|   stm32f401_b_c_lqfp64 IBIS Model
[IBIS ver]   4.2
[File name]  stm32f401_b_c_lqfp64.ibs
[File Rev]   1.0
[Date]   09-06-2015
[Source] Data Created at STMicroelectronics
[Notes]   File originated from ELDO simulations.
[Disclaimer]  This information is for modeling purpose only and is
   not guaranted. The information is subject to change without
   notice.
[Copyright] Copyright 2015 STMicroelectronics Inc.
[Component] stm32f401_b_c_lqfp64
[Manufacturer] STMicroelectronics
[Package]
| variable   typ   min   max
R_pkg   0.0   NA   NA
L_pkg   0.0H   NA   NA
C_pkg   0.0F   NA   NA
[Pin]   signal_name   model_name   R_pin   L_pin   C_pin
1 VBAT POWER 63.756E-3 3.679E-9 93.469E-15
2 PC13-ANTI_TAMP io8p_arwsudq_ft_v33 68.980E-3 4.220E-9 120.000E-15
3 PC14-OSC32_IN io8p_arwsudq_ft 59.336E-3 3.221E-9 71.020E-15
4 PC15-OSC32_OUT io8p_arsudq_ft 55.719E-3 2.846E-9 52.653E-15
5 PH0-OSC_IN io8p_arsudq_ft 52.907E-3 2.555E-9 38.367E-15
6 PH1-OSC_OUT io8p_arsudq_ft 50.897E-3 2.347E-9 28.163E-15
7 NRST ioreset_ft_v33 49.692E-3 2.222E-9 22.041E-15
8 PC0 io8p_arwsudq_ft 49.290E-3 2.180E-9 20.000E-15
9 PC1 io8p_arwsudq_ft 49.290E-3 2.180E-9 20.000E-15
10 PC2 io8p_arwsudq_ft 49.692E-3 2.222E-9 22.041E-15
11 PC3 io8p_arwsudq_ft 50.897E-3 2.347E-9 28.163E-15
12 VSSA GND 52.907E-3 2.555E-9 38.367E-15
13 VDDA POWER 55.719E-3 2.846E-9 52.653E-15
14 PA0-WKUP io8p_arwsudq_ft_v33 59.336E-3 3.221E-9 71.020E-15
15 PA1 io8p_arwsudq_ft 63.756E-3 3.679E-9 93.469E-15
16 PA2 io8p_arwsudq_ft 68.980E-3 4.220E-9 120.000E-15
17 PA3 io8p_arwsudq_ft 68.980E-3 4.220E-9 120.000E-15
18 VSS GND 63.756E-3 3.679E-9 93.469E-15
19 VDD POWER 59.336E-3 3.221E-9 71.020E-15
20 PA4 io8p_ar3wsudq_ft 55.719E-3 2.846E-9 52.653E-15
21 PA5 io8p_ar3wsudq_ft 52.907E-3 2.555E-9 38.367E-15
22 PA6 io8p_ar3wsudq_ft 50.897E-3 2.347E-9 28.163E-15
23 PA7 io8p_arwsudq_ft 49.692E-3 2.222E-9 22.041E-15
24 PC4 io8p_arwsudq_ft 49.290E-3 2.180E-9 20.000E-15
25 PC5 io8p_arwsudq_ft 49.290E-3 2.180E-9 20.000E-15
26 PB0 io8p_ar3wsudq_ft 49.692E-3 2.222E-9 22.041E-15
27 PB1 io8p_ar3wsudq_ft 50.897E-3 2.347E-9 28.163E-15
28 PB2 io8p_arwsudq_ft 52.907E-3 2.555E-9 38.367E-15
29 PB10 io8p_arsudq_i2cin_ft 55.719E-3 2.846E-9 52.653E-15
30 VCAP1 POWER 59.336E-3 3.221E-9 71.020E-15
31 VSS GND 63.756E-3 3.679E-9 93.469E-15
32 VDD POWER 68.980E-3 4.220E-9 120.000E-15
33 PB12 io8p_arsudq_ft 68.980E-3 4.220E-9 120.000E-15
34 PB13 io8p_arsudq_ft 63.756E-3 3.679E-9 93.469E-15
35 PB14 io8p_arsudq_ft 59.336E-3 3.221E-9 71.020E-15
36 PB15 io8p_arsudq_ft 55.719E-3 2.846E-9 52.653E-15
37 PC6 io8p_arsudq_ft 52.907E-3 2.555E-9 38.367E-15
38 PC7 io8p_arsudq_ft 50.897E-3 2.347E-9 28.163E-15
39 PC8 io8p_arsudq_ft 49.692E-3 2.222E-9 22.041E-15
40 PC9 io8p_arsudq_i2cin_ft 49.290E-3 2.180E-9 20.000E-15
41 PA8 io8p_arsudq_i2cin_ft 49.290E-3 2.180E-9 20.000E-15
42 PA9 io8usb_vbus_otg_ft 49.692E-3 2.222E-9 22.041E-15
43 PA10 io8usb_id_otg_ft 50.897E-3 2.347E-9 28.163E-15
44 PA11 io8usb_lsfs_otg_ft 52.907E-3 2.555E-9 38.367E-15
45 PA12 io8usb_lsfs_otg_ft 55.719E-3 2.846E-9 52.653E-15
46 PA13 io8p_arsudq_ft 59.336E-3 3.221E-9 71.020E-15
47 VSS GND 63.756E-3 3.679E-9 93.469E-15
48 VDD POWER 68.980E-3 4.220E-9 120.000E-15
49 PA14 io8p_arsudq_ft 68.980E-3 4.220E-9 120.000E-15
50 PA15 io8p_arsudq_ft 63.756E-3 3.679E-9 93.469E-15
51 PC10 io8p_arsudq_ft 59.336E-3 3.221E-9 71.020E-15
52 PC11 io8p_arsudq_ft 55.719E-3 2.846E-9 52.653E-15
53 PC12 io8p_arsudq_ft 52.907E-3 2.555E-9 38.367E-15
54 PD2 io8p_arsudq_ft 50.897E-3 2.347E-9 28.163E-15
55 PB3 io8p_arsudq_i2cin_ft 49.692E-3 2.222E-9 22.041E-15
56 PB4 io8p_arsudq_i2cin_ft 49.290E-3 2.180E-9 20.000E-15
57 PB5 io8p_ar3wsudq_ft 49.290E-3 2.180E-9 20.000E-15
58 PB6 io8p_arsudq_i2cin_ft 49.692E-3 2.222E-9 22.041E-15
59 PB7 io8p_arsudq_i2cin_ft 50.897E-3 2.347E-9 28.163E-15
60 BOOT0 vpp_test_hv 52.907E-3 2.555E-9 38.367E-15
61 PB8 io8p_arsudq_i2cin_ft 55.719E-3 2.846E-9 52.653E-15
62 PB9 io8p_arsudq_i2cin_ft 59.336E-3 3.221E-9 71.020E-15
63 VSS GND 63.756E-3 3.679E-9 93.469E-15
64 VDD POWER 68.980E-3 4.220E-9 120.000E-15
[Diff Pin]   inv_pin   vdiff   tdelay_typ  tdelay_min  tdelay_max
44 45 200mV   NA   NA   NA
[Model Selector] io8p_ar3wsudq_ft
io8p00_ar3wsudq_ft_pd_lv  "SPEED00 1P8V, PD=40kOhm"
io8p00_ar3wsudq_ft_pu_lv  "SPEED00 1P8V, PU=40kOhm"
io8p00_ar3wsudq_ft_lv  "SPEED00 1P8V"
io8p01_ar3wsudq_ft_pd_lv  "SPEED01 1P8V, PD=40kOhm"
io8p01_ar3wsudq_ft_pu_lv  "SPEED01 1P8V, PU=40kOhm"
io8p01_ar3wsudq_ft_lv  "SPEED01 1P8V"
io8p10_ar3wsudq_ft_pd_lv  "SPEED10 1P8V, PD=40kOhm"
io8p10_ar3wsudq_ft_pu_lv  "SPEED10 1P8V, PU=40kOhm"
io8p10_ar3wsudq_ft_lv  "SPEED10 1P8V"
io8p11_ar3wsudq_ft_pd_lv  "SPEED11 1P8V, PD=40kOhm"
io8p11_ar3wsudq_ft_pu_lv  "SPEED11 1P8V, PU=40kOhm"
io8p11_ar3wsudq_ft_lv  "SPEED11 1P8V"
io8p00_ar3wsudq_ft_pd  "SPEED00, PD=40kOhm"
io8p00_ar3wsudq_ft_pu  "SPEED00, PU=40kOhm"
io8p00_ar3wsudq_ft  "SPEED00"
io8p01_ar3wsudq_ft_pd  "SPEED01, PD=40kOhm"
io8p01_ar3wsudq_ft_pu  "SPEED01, PU=40kOhm"
io8p01_ar3wsudq_ft  "SPEED01"
io8p10_ar3wsudq_ft_pd  "SPEED10, PD=40kOhm"
io8p10_ar3wsudq_ft_pu  "SPEED10, PU=40kOhm"
io8p10_ar3wsudq_ft  "SPEED10"
io8p11_ar3wsudq_ft_pd  "SPEED11, PD=40kOhm"
io8p11_ar3wsudq_ft_pu  "SPEED11, PU=40kOhm"
io8p11_ar3wsudq_ft  "SPEED11"
[Model Selector] io8p_arsudq_ft
io8p00_arsudq_ft_pd_lv  "SPEED00 1P8V, PD=40kOhm"
io8p00_arsudq_ft_pu_lv  "SPEED00 1P8V, PU=40kOhm"
io8p00_arsudq_ft_lv  "SPEED00 1P8V"
io8p01_arsudq_ft_pd_lv  "SPEED01 1P8V, PD=40kOhm"
io8p01_arsudq_ft_pu_lv  "SPEED01 1P8V, PU=40kOhm"
io8p01_arsudq_ft_lv  "SPEED01 1P8V"
io8p10_arsudq_ft_pd_lv  "SPEED10 1P8V, PD=40kOhm"
io8p10_arsudq_ft_pu_lv  "SPEED10 1P8V, PU=40kOhm"
io8p10_arsudq_ft_lv  "SPEED10 1P8V"
io8p11_arsudq_ft_pd_lv  "SPEED11 1P8V, PD=40kOhm"
io8p11_arsudq_ft_pu_lv  "SPEED11 1P8V, PU=40kOhm"
io8p11_arsudq_ft_lv  "SPEED11 1P8V"
io8p00_arsudq_ft_pd  "SPEED00, PD=40kOhm"
io8p00_arsudq_ft_pu  "SPEED00, PU=40kOhm"
io8p00_arsudq_ft  "SPEED00"
io8p01_arsudq_ft_pd  "SPEED01, PD=40kOhm"
io8p01_arsudq_ft_pu  "SPEED01, PU=40kOhm"
io8p01_arsudq_ft  "SPEED01"
io8p10_arsudq_ft_pd  "SPEED10, PD=40kOhm"
io8p10_arsudq_ft_pu  "SPEED10, PU=40kOhm"
io8p10_arsudq_ft  "SPEED10"
io8p11_arsudq_ft_pd  "SPEED11, PD=40kOhm"
io8p11_arsudq_ft_pu  "SPEED11, PU=40kOhm"
io8p11_arsudq_ft  "SPEED11"
[Model Selector] io8p_arsudq_i2cin_ft
io8p00_arsudq_i2cin_ft_pd_lv  "SPEED00 1P8V, PD=40kOhm"
io8p00_arsudq_i2cin_ft_pu_lv  "SPEED00 1P8V, PU=40kOhm"
io8p00_arsudq_i2cin_ft_lv  "SPEED00 1P8V"
io8p01_arsudq_i2cin_ft_pd_lv  "SPEED01 1P8V, PD=40kOhm"
io8p01_arsudq_i2cin_ft_pu_lv  "SPEED01 1P8V, PU=40kOhm"
io8p01_arsudq_i2cin_ft_lv  "SPEED01 1P8V"
io8p10_arsudq_i2cin_ft_pd_lv  "SPEED10 1P8V, PD=40kOhm"
io8p10_arsudq_i2cin_ft_pu_lv  "SPEED10 1P8V, PU=40kOhm"
io8p10_arsudq_i2cin_ft_lv  "SPEED10 1P8V"
io8p11_arsudq_i2cin_ft_pd_lv  "SPEED11 1P8V, PD=40kOhm"
io8p11_arsudq_i2cin_ft_pu_lv  "SPEED11 1P8V, PU=40kOhm"
io8p11_arsudq_i2cin_ft_lv  "SPEED11 1P8V"
io8p00_arsudq_i2cin_ft_pd  "SPEED00, PD=40kOhm"
io8p00_arsudq_i2cin_ft_pu  "SPEED00, PU=40kOhm"
io8p00_arsudq_i2cin_ft  "SPEED00"
io8p01_arsudq_i2cin_ft_pd  "SPEED01, PD=40kOhm"
io8p01_arsudq_i2cin_ft_pu  "SPEED01, PU=40kOhm"
io8p01_arsudq_i2cin_ft  "SPEED01"
io8p10_arsudq_i2cin_ft_pd  "SPEED10, PD=40kOhm"
io8p10_arsudq_i2cin_ft_pu  "SPEED10, PU=40kOhm"
io8p10_arsudq_i2cin_ft  "SPEED10"
io8p11_arsudq_i2cin_ft_pd  "SPEED11, PD=40kOhm"
io8p11_arsudq_i2cin_ft_pu  "SPEED11, PU=40kOhm"
io8p11_arsudq_i2cin_ft  "SPEED11"
[Model Selector] io8p_arwsudq_ft
io8p00_arwsudq_ft_pd_lv  "SPEED00 1P8V, PD=40kOhm"
io8p00_arwsudq_ft_pu_lv  "SPEED00 1P8V, PU=40kOhm"
io8p00_arwsudq_ft_lv  "SPEED00 1P8V"
io8p01_arwsudq_ft_pd_lv  "SPEED01 1P8V, PD=40kOhm"
io8p01_arwsudq_ft_pu_lv  "SPEED01 1P8V, PU=40kOhm"
io8p01_arwsudq_ft_lv  "SPEED01 1P8V"
io8p10_arwsudq_ft_pd_lv  "SPEED10 1P8V, PD=40kOhm"
io8p10_arwsudq_ft_pu_lv  "SPEED10 1P8V, PU=40kOhm"
io8p10_arwsudq_ft_lv  "SPEED10 1P8V"
io8p11_arwsudq_ft_pd_lv  "SPEED11 1P8V, PD=40kOhm"
io8p11_arwsudq_ft_pu_lv  "SPEED11 1P8V, PU=40kOhm"
io8p11_arwsudq_ft_lv  "SPEED11 1P8V"
io8p00_arwsudq_ft_pd  "SPEED00, PD=40kOhm"
io8p00_arwsudq_ft_pu  "SPEED00, PU=40kOhm"
io8p00_arwsudq_ft  "SPEED00"
io8p01_arwsudq_ft_pd  "SPEED01, PD=40kOhm"
io8p01_arwsudq_ft_pu  "SPEED01, PU=40kOhm"
io8p01_arwsudq_ft  "SPEED01"
io8p10_arwsudq_ft_pd  "SPEED10, PD=40kOhm"
io8p10_arwsudq_ft_pu  "SPEED10, PU=40kOhm"
io8p10_arwsudq_ft  "SPEED10"
io8p11_arwsudq_ft_pd  "SPEED11, PD=40kOhm"
io8p11_arwsudq_ft_pu  "SPEED11, PU=40kOhm"
io8p11_arwsudq_ft  "SPEED11"
[Model Selector] io8p_arwsudq_ft_v33
io8p00_arwsudq_ft_v33_pd_lv  "SPEED00 1P8V, PD=40kOhm"
io8p00_arwsudq_ft_v33_pu_lv  "SPEED00 1P8V, PU=40kOhm"
io8p00_arwsudq_ft_v33_lv  "SPEED00 1P8V"
io8p01_arwsudq_ft_v33_pd_lv  "SPEED01 1P8V, PD=40kOhm"
io8p01_arwsudq_ft_v33_pu_lv  "SPEED01 1P8V, PU=40kOhm"
io8p01_arwsudq_ft_v33_lv  "SPEED01 1P8V"
io8p10_arwsudq_ft_v33_pd_lv  "SPEED10 1P8V, PD=40kOhm"
io8p10_arwsudq_ft_v33_pu_lv  "SPEED10 1P8V, PU=40kOhm"
io8p10_arwsudq_ft_v33_lv  "SPEED10 1P8V"
io8p11_arwsudq_ft_v33_pd_lv  "SPEED11 1P8V, PD=40kOhm"
io8p11_arwsudq_ft_v33_pu_lv  "SPEED11 1P8V, PU=40kOhm"
io8p11_arwsudq_ft_v33_lv  "SPEED11 1P8V"
io8p00_arwsudq_ft_v33_pd  "SPEED00, PD=40kOhm"
io8p00_arwsudq_ft_v33_pu  "SPEED00, PU=40kOhm"
io8p00_arwsudq_ft_v33  "SPEED00"
io8p01_arwsudq_ft_v33_pd  "SPEED01, PD=40kOhm"
io8p01_arwsudq_ft_v33_pu  "SPEED01, PU=40kOhm"
io8p01_arwsudq_ft_v33  "SPEED01"
io8p10_arwsudq_ft_v33_pd  "SPEED10, PD=40kOhm"
io8p10_arwsudq_ft_v33_pu  "SPEED10, PU=40kOhm"
io8p10_arwsudq_ft_v33  "SPEED10"
io8p11_arwsudq_ft_v33_pd  "SPEED11, PD=40kOhm"
io8p11_arwsudq_ft_v33_pu  "SPEED11, PU=40kOhm"
io8p11_arwsudq_ft_v33  "SPEED11"
[Model Selector] io8usb_id_otg_ft
io8p00_id_otg_ft_pd_lv  "SPEED00 1P8V, PD=14kOhm"
io8p00_id_otg_ft_pu_lv  "SPEED00 1P8V, PU=14kOhm"
io8p00_id_otg_ft_lv  "SPEED00 1P8V"
io8p01_id_otg_ft_pd_lv  "SPEED01 1P8V, PD=14kOhm"
io8p01_id_otg_ft_pu_lv  "SPEED01 1P8V, PU=14kOhm"
io8p01_id_otg_ft_lv  "SPEED01 1P8V"
io8p10_id_otg_ft_pd_lv  "SPEED10 1P8V, PD=14kOhm"
io8p10_id_otg_ft_pu_lv  "SPEED10 1P8V, PU=14kOhm"
io8p10_id_otg_ft_lv  "SPEED10 1P8V"
io8p11_id_otg_ft_pd_lv  "SPEED11 1P8V, PD=14kOhm"
io8p11_id_otg_ft_pu_lv  "SPEED11 1P8V, PU=14kOhm"
io8p11_id_otg_ft_lv  "SPEED11 1P8V"
io8p00_id_otg_ft_pd  "SPEED00, PD=14kOhm"
io8p00_id_otg_ft_pu  "SPEED00, PU=14kOhm"
io8p00_id_otg_ft  "SPEED00"
io8p01_id_otg_ft_pd  "SPEED01, PD=14kOhm"
io8p01_id_otg_ft_pu  "SPEED01, PU=14kOhm"
io8p01_id_otg_ft  "SPEED01"
io8p10_id_otg_ft_pd  "SPEED10, PD=14kOhm"
io8p10_id_otg_ft_pu  "SPEED10, PU=14kOhm"
io8p10_id_otg_ft  "SPEED10"
io8p11_id_otg_ft_pd  "SPEED11, PD=14kOhm"
io8p11_id_otg_ft_pu  "SPEED11, PU=14kOhm"
io8p11_id_otg_ft  "SPEED11"
[Model Selector] io8usb_lsfs_otg_ft
io8usb_ls_otg_ft_dpdn_pd  "LS USB DP/DN IO + PD=20kOhm"
io8usb_ls_otg_ft_dpdn_pupu2  "LS USB DP/DN IO + PU/PU2=2.2kOhm"
io8usb_ls_otg_ft_dpdn_pu2  "LS USB DP/DN IO + PU2=1.2kOhm"
io8usb_ls_otg_ft_dpdn_pu  "LS USB DP/DN IO + PU=1.2kOhm"
io8usb_ls_otg_ft_dpdn  "LS USB DP/DN IO"
io8usb_fs_otg_ft_dpdn_pd  "HS USB DP/DN IO + PD=20kOhm"
io8usb_fs_otg_ft_dpdn_pupu2  "HS USB DP/DN IO + PU/PU2=2.2kOhm"
io8usb_fs_otg_ft_dpdn_pu2  "HS USB DP/DN IO + PU2=1.2kOhm"
io8usb_fs_otg_ft_dpdn_pu  "HS USB DP/DN IO + PU=1.2kOhm"
io8usb_fs_otg_ft_dpdn  "HS USB DP/DN IO"
io8p00_lsfs_otg_ft_pd_lv  "SPEED00 1P8V, PD=40kOhm"
io8p00_lsfs_otg_ft_pu_lv  "SPEED00 1P8V, PU=40kOhm"
io8p00_lsfs_otg_ft_lv  "SPEED00 1P8V"
io8p01_lsfs_otg_ft_pd_lv  "SPEED01 1P8V, PD=40kOhm"
io8p01_lsfs_otg_ft_pu_lv  "SPEED01 1P8V, PU=40kOhm"
io8p01_lsfs_otg_ft_lv  "SPEED01 1P8V"
io8p10_lsfs_otg_ft_pd_lv  "SPEED10 1P8V, PD=40kOhm"
io8p10_lsfs_otg_ft_pu_lv  "SPEED10 1P8V, PU=40kOhm"
io8p10_lsfs_otg_ft_lv  "SPEED10 1P8V"
io8p11_lsfs_otg_ft_pd_lv  "SPEED11 1P8V, PD=40kOhm"
io8p11_lsfs_otg_ft_pu_lv  "SPEED11 1P8V, PU=40kOhm"
io8p11_lsfs_otg_ft_lv  "SPEED11 1P8V"
io8p00_lsfs_otg_ft_pd  "SPEED00, PD=40kOhm"
io8p00_lsfs_otg_ft_pu  "SPEED00, PU=40kOhm"
io8p00_lsfs_otg_ft  "SPEED00"
io8p01_lsfs_otg_ft_pd  "SPEED01, PD=40kOhm"
io8p01_lsfs_otg_ft_pu  "SPEED01, PU=40kOhm"
io8p01_lsfs_otg_ft  "SPEED01"
io8p10_lsfs_otg_ft_pd  "SPEED10, PD=40kOhm"
io8p10_lsfs_otg_ft_pu  "SPEED10, PU=40kOhm"
io8p10_lsfs_otg_ft  "SPEED10"
io8p11_lsfs_otg_ft_pd  "SPEED11, PD=40kOhm"
io8p11_lsfs_otg_ft_pu  "SPEED11, PU=40kOhm"
io8p11_lsfs_otg_ft  "SPEED11"
[Model Selector] io8usb_vbus_otg_ft
io8psenb_vbus_otg_ft  "VBUS PULSE, SENSE VB"
io8psenab_vbus_otg_ft  "VBUS PULSE, SENSE VA and VB"
io8psena_vbus_otg_ft  "VBUS PULSE, SENSE VA"
io8psen_vbus_otg_ft  "VBUS PULSE"
io8p00_vbus_otg_ft_pd_lv  "SPEED00 1P8V, PD=40kOhm"
io8p00_vbus_otg_ft_pu_lv  "SPEED00 1P8V, PU=40kOhm"
io8p00_vbus_otg_ft_lv  "SPEED00 1P8V"
io8p01_vbus_otg_ft_pd_lv  "SPEED01 1P8V, PD=40kOhm"
io8p01_vbus_otg_ft_pu_lv  "SPEED01 1P8V, PU=40kOhm"
io8p01_vbus_otg_ft_lv  "SPEED01 1P8V"
io8p10_vbus_otg_ft_pd_lv  "SPEED10 1P8V, PD=40kOhm"
io8p10_vbus_otg_ft_pu_lv  "SPEED10 1P8V, PU=40kOhm"
io8p10_vbus_otg_ft_lv  "SPEED10 1P8V"
io8p11_vbus_otg_ft_pd_lv  "SPEED11 1P8V, PD=40kOhm"
io8p11_vbus_otg_ft_pu_lv  "SPEED11 1P8V, PU=40kOhm"
io8p11_vbus_otg_ft_lv  "SPEED11 1P8V"
io8p00_vbus_otg_ft_pd  "SPEED00, PD=40kOhm"
io8p00_vbus_otg_ft_pu  "SPEED00, PU=40kOhm"
io8p00_vbus_otg_ft  "SPEED00"
io8p01_vbus_otg_ft_pd  "SPEED01, PD=40kOhm"
io8p01_vbus_otg_ft_pu  "SPEED01, PU=40kOhm"
io8p01_vbus_otg_ft  "SPEED01"
io8p10_vbus_otg_ft_pd  "SPEED10, PD=40kOhm"
io8p10_vbus_otg_ft_pu  "SPEED10, PU=40kOhm"
io8p10_vbus_otg_ft  "SPEED10"
io8p11_vbus_otg_ft_pd  "SPEED11, PD=40kOhm"
io8p11_vbus_otg_ft_pu  "SPEED11, PU=40kOhm"
io8p11_vbus_otg_ft  "SPEED11"
[Model Selector] ioreset_ft_v33
ioreset_ft_v33_pu_lv  "ioreset 1P8V + PU=40kOhm"
ioreset_ft_v33_nopu_lv  "ioreset 1P8V"
ioreset_ft_v33_pu  "ioreset + PU=40kOhm"
ioreset_ft_v33_nopu  "ioreset"
[Model Selector] vpp_test_hv
vpp_test_hv_2p4  "Input Buffer 1P8V"
vpp_test_hv_3p3  "Input Buffer"
| Models and submodels in the file (212): io8p00_ar3wsudq_ft_pd_lv (I/O), io8p00_ar3wsudq_ft_pu_lv (I/O), io8p00_ar3wsudq_ft_lv (I/O), io8p01_ar3wsudq_ft_pd_lv (I/O), io8p01_ar3wsudq_ft_pu_lv (I/O), io8p01_ar3wsudq_ft_lv (I/O), io8p10_ar3wsudq_ft_pd_lv (I/O), io8p10_ar3wsudq_ft_pu_lv (I/O), io8p10_ar3wsudq_ft_lv (I/O), io8p11_ar3wsudq_ft_pd_lv (I/O), io8p11_ar3wsudq_ft_pu_lv (I/O), io8p11_ar3wsudq_ft_lv (I/O), io8p00_ar3wsudq_ft_pd (I/O), io8p00_ar3wsudq_ft_pu (I/O), io8p00_ar3wsudq_ft (I/O), io8p01_ar3wsudq_ft_pd (I/O), io8p01_ar3wsudq_ft_pu (I/O), io8p01_ar3wsudq_ft (I/O), io8p10_ar3wsudq_ft_pd (I/O), io8p10_ar3wsudq_ft_pu (I/O), io8p10_ar3wsudq_ft (I/O), io8p11_ar3wsudq_ft_pd (I/O), io8p11_ar3wsudq_ft_pu (I/O), io8p11_ar3wsudq_ft (I/O), io8p00_arsudq_ft_pd_lv (I/O), io8p00_arsudq_ft_pu_lv (I/O), io8p00_arsudq_ft_lv (I/O), io8p01_arsudq_ft_pd_lv (I/O), io8p01_arsudq_ft_pu_lv (I/O), io8p01_arsudq_ft_lv (I/O), io8p10_arsudq_ft_pd_lv (I/O), io8p10_arsudq_ft_pu_lv (I/O), io8p10_arsudq_ft_lv (I/O), io8p11_arsudq_ft_pd_lv (I/O), io8p11_arsudq_ft_pu_lv (I/O), io8p11_arsudq_ft_lv (I/O), io8p00_arsudq_ft_pd (I/O), io8p00_arsudq_ft_pu (I/O), io8p00_arsudq_ft (I/O), io8p01_arsudq_ft_pd (I/O), io8p01_arsudq_ft_pu (I/O), io8p01_arsudq_ft (I/O), io8p10_arsudq_ft_pd (I/O), io8p10_arsudq_ft_pu (I/O), io8p10_arsudq_ft (I/O), io8p11_arsudq_ft_pd (I/O), io8p11_arsudq_ft_pu (I/O), io8p11_arsudq_ft (I/O), io8p00_arsudq_i2cin_ft_pd_lv (I/O), io8p00_arsudq_i2cin_ft_pu_lv (I/O), io8p00_arsudq_i2cin_ft_lv (I/O), io8p01_arsudq_i2cin_ft_pd_lv (I/O), io8p01_arsudq_i2cin_ft_pu_lv (I/O), io8p01_arsudq_i2cin_ft_lv (I/O), io8p10_arsudq_i2cin_ft_pd_lv (I/O), io8p10_arsudq_i2cin_ft_pu_lv (I/O), io8p10_arsudq_i2cin_ft_lv (I/O), io8p11_arsudq_i2cin_ft_pd_lv (I/O), io8p11_arsudq_i2cin_ft_pu_lv (I/O), io8p11_arsudq_i2cin_ft_lv (I/O), io8p00_arsudq_i2cin_ft_pd (I/O), io8p00_arsudq_i2cin_ft_pu (I/O), io8p00_arsudq_i2cin_ft (I/O), io8p01_arsudq_i2cin_ft_pd (I/O), io8p01_arsudq_i2cin_ft_pu (I/O), io8p01_arsudq_i2cin_ft (I/O), io8p10_arsudq_i2cin_ft_pd (I/O), io8p10_arsudq_i2cin_ft_pu (I/O), io8p10_arsudq_i2cin_ft (I/O), io8p11_arsudq_i2cin_ft_pd (I/O), io8p11_arsudq_i2cin_ft_pu (I/O), io8p11_arsudq_i2cin_ft (I/O), io8p00_arwsudq_ft_pd_lv (I/O), io8p00_arwsudq_ft_pu_lv (I/O), io8p00_arwsudq_ft_lv (I/O), io8p01_arwsudq_ft_pd_lv (I/O), io8p01_arwsudq_ft_pu_lv (I/O), io8p01_arwsudq_ft_lv (I/O), io8p10_arwsudq_ft_pd_lv (I/O), io8p10_arwsudq_ft_pu_lv (I/O)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
